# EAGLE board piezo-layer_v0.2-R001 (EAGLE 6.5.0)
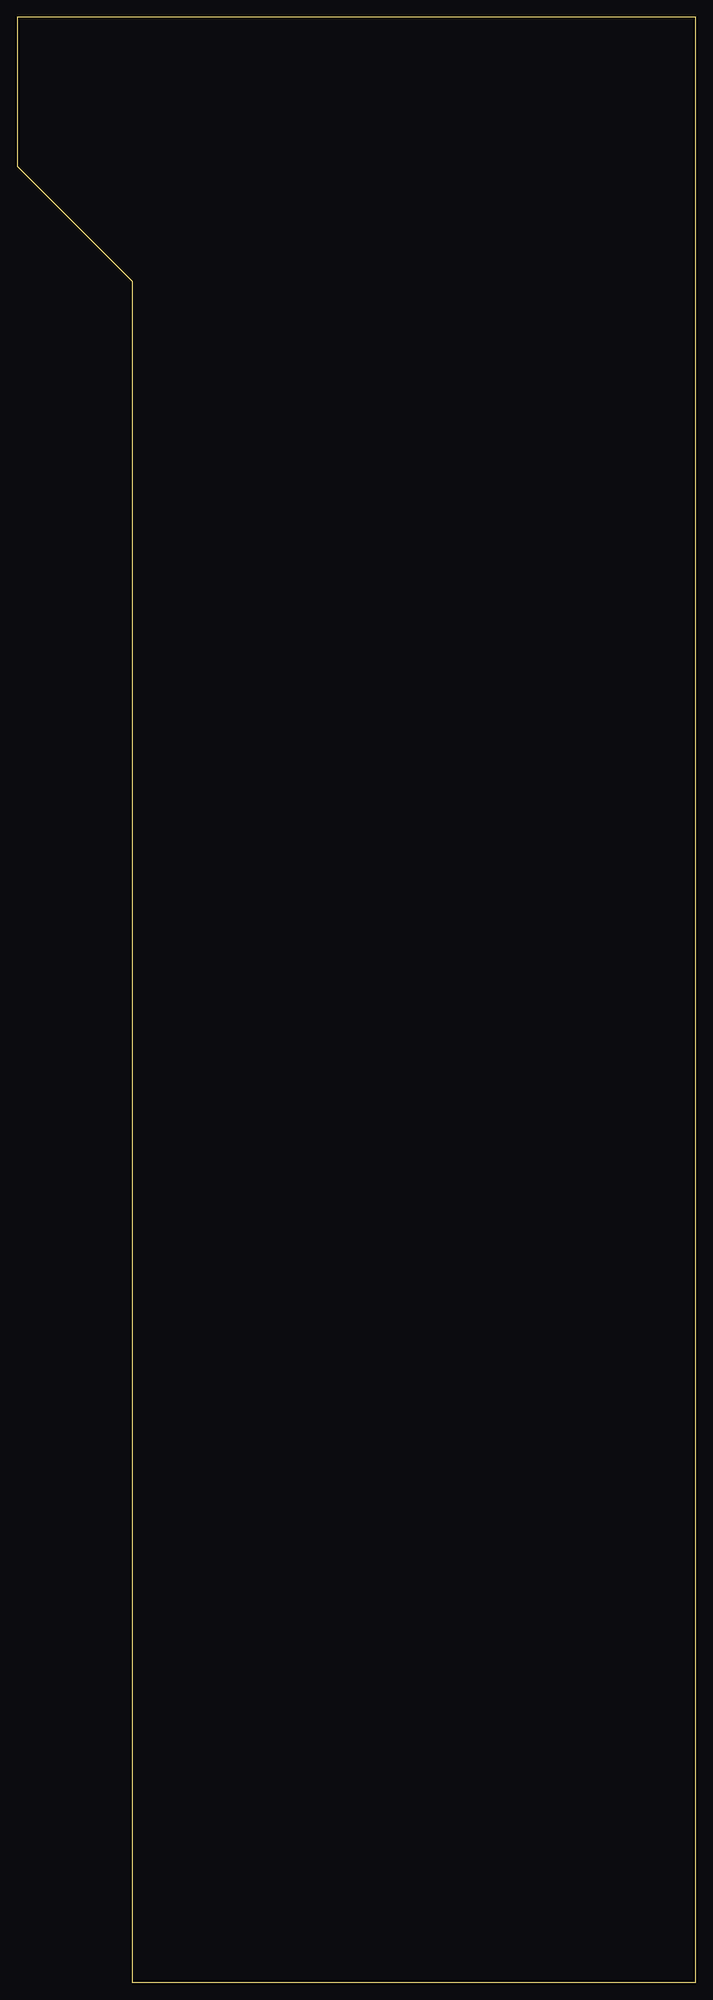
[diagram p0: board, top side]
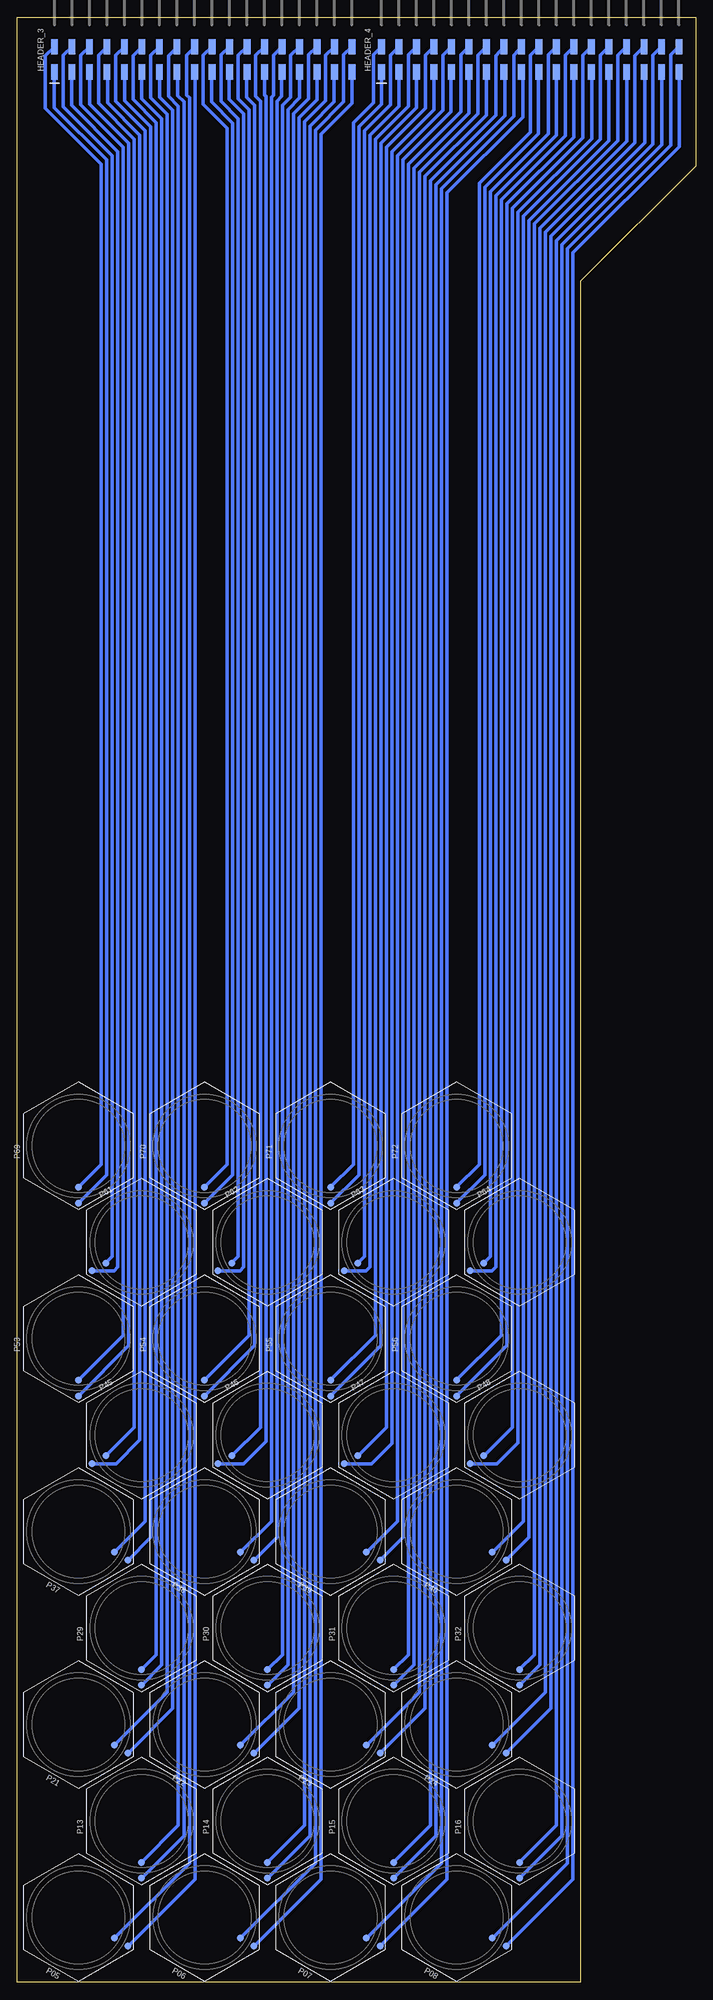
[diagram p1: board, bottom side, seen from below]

Size 98.5 x 285.2 mm. Coordinates in mm from the lower left corner, seen from the top.
Outline: 16.7,0 98.5,0 98.5,285.2 0,285.2 0,263.6 16.7,246.9 16.7,0
Copper layers (1*16): Top 0.009mm / dielectric 0.2mm / Bottom 0.018mm
Design rules "1L-0.2-0.15_0.3mm *": minimum track width 0.2mm, minimum drill 0.3mm, track to track 0.15mm, track to pad 0.15mm, pad to pad 0.15mm, via to via 0.15mm, smd to smd 0.15mm, copper to edge 0.5mm, drill to drill 1mm, minimum pad ring 10mil, minimum via ring 8mil, stop-mask expansion 4mil, vias tented up to drill 0mil, thermal gap 10mil

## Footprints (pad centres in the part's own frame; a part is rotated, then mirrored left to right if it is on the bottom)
2X18_2.54_90_SMD = smd 1 x 2.2: 1 -21.59,-1.84; 2 -21.59,1.84; 3 -19.05,-1.84; 4 -19.05,1.84; 5 -16.51,-1.84; 6 -16.51,1.84; 7 -13.97,-1.84; 8 -13.97,1.84; 9 -11.43,-1.84; 10 -11.43,1.84; 11 -8.89,-1.84; 12 -8.89,1.84; 13 -6.35,-1.84; 14 -6.35,1.84; 15 -3.81,-1.84; 16 -3.81,1.84; 17 -1.27,-1.84; 18 -1.27,1.84; 19 1.27,-1.84; 20 1.27,1.84; 21 3.81,-1.84; 22 3.81,1.84; 23 6.35,-1.84; 24 6.35,1.84; 25 8.89,-1.84; 26 8.89,1.84; 27 11.43,-1.84; 28 11.43,1.84; 29 13.97,-1.84; 30 13.97,1.84; 31 16.51,-1.84; 32 16.51,1.84; 33 19.05,-1.84; 34 19.05,1.84; 35 21.59,-1.84; 36 21.59,1.84
PIEZO-BENDER-HEX_16MM_1+_1- = smd 1 x 1: PAD1 -8.3,0; TIP1 -6,0

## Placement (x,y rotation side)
HEADER_3  HEADER_2X18-2.54_90_SMD  [2X18_2.54_90_SMD]  71.5,279.1 0 bottom
HEADER_4  HEADER_2X18-2.54_90_SMD  [2X18_2.54_90_SMD]  24,279.1 0 bottom
P05  PIEZO-BENDER-HEX_1-1  [PIEZO-BENDER-HEX_16MM_1+_1-]  89.6,9.4 150 bottom
P06  PIEZO-BENDER-HEX_1-1  [PIEZO-BENDER-HEX_16MM_1+_1-]  71.3,9.4 150 bottom
P07  PIEZO-BENDER-HEX_1-1  [PIEZO-BENDER-HEX_16MM_1+_1-]  53,9.4 150 bottom
P08  PIEZO-BENDER-HEX_1-1  [PIEZO-BENDER-HEX_16MM_1+_1-]  34.7,9.4 150 bottom
P13  PIEZO-BENDER-HEX_1-1  [PIEZO-BENDER-HEX_16MM_1+_1-]  80.45,23.4 90 bottom
P14  PIEZO-BENDER-HEX_1-1  [PIEZO-BENDER-HEX_16MM_1+_1-]  62.15,23.4 90 bottom
P15  PIEZO-BENDER-HEX_1-1  [PIEZO-BENDER-HEX_16MM_1+_1-]  43.85,23.4 90 bottom
P16  PIEZO-BENDER-HEX_1-1  [PIEZO-BENDER-HEX_16MM_1+_1-]  25.55,23.4 90 bottom
P21  PIEZO-BENDER-HEX_1-1  [PIEZO-BENDER-HEX_16MM_1+_1-]  89.6,37.4 150 bottom
P22  PIEZO-BENDER-HEX_1-1  [PIEZO-BENDER-HEX_16MM_1+_1-]  71.3,37.4 150 bottom
P23  PIEZO-BENDER-HEX_1-1  [PIEZO-BENDER-HEX_16MM_1+_1-]  53,37.4 150 bottom
P24  PIEZO-BENDER-HEX_1-1  [PIEZO-BENDER-HEX_16MM_1+_1-]  34.7,37.4 150 bottom
P29  PIEZO-BENDER-HEX_1-1  [PIEZO-BENDER-HEX_16MM_1+_1-]  80.45,51.4 90 bottom
P30  PIEZO-BENDER-HEX_1-1  [PIEZO-BENDER-HEX_16MM_1+_1-]  62.15,51.4 90 bottom
P31  PIEZO-BENDER-HEX_1-1  [PIEZO-BENDER-HEX_16MM_1+_1-]  43.85,51.4 90 bottom
P32  PIEZO-BENDER-HEX_1-1  [PIEZO-BENDER-HEX_16MM_1+_1-]  25.55,51.4 90 bottom
P37  PIEZO-BENDER-HEX_1-1  [PIEZO-BENDER-HEX_16MM_1+_1-]  89.6,65.4 150 bottom
P38  PIEZO-BENDER-HEX_1-1  [PIEZO-BENDER-HEX_16MM_1+_1-]  71.3,65.4 150 bottom
P39  PIEZO-BENDER-HEX_1-1  [PIEZO-BENDER-HEX_16MM_1+_1-]  53,65.4 150 bottom
P40  PIEZO-BENDER-HEX_1-1  [PIEZO-BENDER-HEX_16MM_1+_1-]  34.7,65.4 150 bottom
P45  PIEZO-BENDER-HEX_1-1  [PIEZO-BENDER-HEX_16MM_1+_1-]  80.45,79.4 30 bottom
P46  PIEZO-BENDER-HEX_1-1  [PIEZO-BENDER-HEX_16MM_1+_1-]  62.15,79.4 30 bottom
P47  PIEZO-BENDER-HEX_1-1  [PIEZO-BENDER-HEX_16MM_1+_1-]  43.85,79.4 30 bottom
P48  PIEZO-BENDER-HEX_1-1  [PIEZO-BENDER-HEX_16MM_1+_1-]  25.55,79.4 30 bottom
P53  PIEZO-BENDER-HEX_1-1  [PIEZO-BENDER-HEX_16MM_1+_1-]  89.6,93.4 90 bottom
P54  PIEZO-BENDER-HEX_1-1  [PIEZO-BENDER-HEX_16MM_1+_1-]  71.3,93.4 90 bottom
P55  PIEZO-BENDER-HEX_1-1  [PIEZO-BENDER-HEX_16MM_1+_1-]  53,93.4 90 bottom
P56  PIEZO-BENDER-HEX_1-1  [PIEZO-BENDER-HEX_16MM_1+_1-]  34.7,93.4 90 bottom
P61  PIEZO-BENDER-HEX_1-1  [PIEZO-BENDER-HEX_16MM_1+_1-]  80.45,107.4 30 bottom
P62  PIEZO-BENDER-HEX_1-1  [PIEZO-BENDER-HEX_16MM_1+_1-]  62.15,107.4 30 bottom
P63  PIEZO-BENDER-HEX_1-1  [PIEZO-BENDER-HEX_16MM_1+_1-]  43.85,107.4 30 bottom
P64  PIEZO-BENDER-HEX_1-1  [PIEZO-BENDER-HEX_16MM_1+_1-]  25.55,107.4 30 bottom
P69  PIEZO-BENDER-HEX_1-1  [PIEZO-BENDER-HEX_16MM_1+_1-]  89.6,121.4 90 bottom
P70  PIEZO-BENDER-HEX_1-1  [PIEZO-BENDER-HEX_16MM_1+_1-]  71.3,121.4 90 bottom
P71  PIEZO-BENDER-HEX_1-1  [PIEZO-BENDER-HEX_16MM_1+_1-]  53,121.4 90 bottom
P72  PIEZO-BENDER-HEX_1-1  [PIEZO-BENDER-HEX_16MM_1+_1-]  34.7,121.4 90 bottom

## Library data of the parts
HEADER_3 HEADER_4 = SABRe
P05-P08 P13-P16 P21-P24 P29-P32 P37-P40 P45-P48 P53-P56 P61-P64 P69-P72 = ICST

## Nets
BUS+5: HEADER_3.18 P05.TIP1
BUS+6: HEADER_3.36 P06.TIP1
BUS+7: HEADER_4.18 P07.TIP1
BUS+8: HEADER_4.36 P08.TIP1
BUS+13: HEADER_3.16 P13.TIP1
BUS+14: HEADER_3.34 P14.TIP1
BUS+15: HEADER_4.16 P15.TIP1
BUS+16: HEADER_4.34 P16.TIP1
BUS+21: HEADER_3.14 P21.TIP1
BUS+22: HEADER_3.32 P22.TIP1
BUS+23: HEADER_4.14 P23.TIP1
BUS+24: HEADER_4.32 P24.TIP1
BUS+29: HEADER_3.12 P29.TIP1
BUS+30: HEADER_3.30 P30.TIP1
BUS+31: HEADER_4.12 P31.TIP1
BUS+32: HEADER_4.30 P32.TIP1
BUS+37: HEADER_3.10 P37.TIP1
BUS+38: HEADER_3.28 P38.TIP1
BUS+39: HEADER_4.10 P39.TIP1
BUS+40: HEADER_4.28 P40.TIP1
BUS+45: HEADER_3.8 P45.TIP1
BUS+46: HEADER_3.26 P46.TIP1
BUS+47: HEADER_4.8 P47.TIP1
BUS+48: HEADER_4.26 P48.TIP1
BUS+53: HEADER_3.6 P53.TIP1
BUS+54: HEADER_3.24 P54.TIP1
BUS+55: HEADER_4.6 P55.TIP1
BUS+56: HEADER_4.24 P56.TIP1
BUS+61: HEADER_3.4 P61.TIP1
BUS+62: HEADER_3.22 P62.TIP1
BUS+63: HEADER_4.4 P63.TIP1
BUS+64: HEADER_4.22 P64.TIP1
BUS+69: HEADER_3.2 P69.TIP1
BUS+70: HEADER_3.20 P70.TIP1
BUS+71: HEADER_4.2 P71.TIP1
BUS+72: HEADER_4.20 P72.TIP1
BUS-5: HEADER_3.17 P05.PAD1
BUS-6: HEADER_3.35 P06.PAD1
BUS-7: HEADER_4.17 P07.PAD1
BUS-8: HEADER_4.35 P08.PAD1
BUS-13: HEADER_3.15 P13.PAD1
BUS-14: HEADER_3.33 P14.PAD1
BUS-15: HEADER_4.15 P15.PAD1
BUS-16: HEADER_4.33 P16.PAD1
BUS-21: HEADER_3.13 P21.PAD1
BUS-22: HEADER_3.31 P22.PAD1
BUS-23: HEADER_4.13 P23.PAD1
BUS-24: HEADER_4.31 P24.PAD1
BUS-29: HEADER_3.11 P29.PAD1
BUS-30: HEADER_3.29 P30.PAD1
BUS-31: HEADER_4.11 P31.PAD1
BUS-32: HEADER_4.29 P32.PAD1
BUS-37: HEADER_3.9 P37.PAD1
BUS-38: HEADER_3.27 P38.PAD1
BUS-39: HEADER_4.9 P39.PAD1
BUS-40: HEADER_4.27 P40.PAD1
BUS-45: HEADER_3.7 P45.PAD1
BUS-46: HEADER_3.25 P46.PAD1
BUS-47: HEADER_4.7 P47.PAD1
BUS-48: HEADER_4.25 P48.PAD1
BUS-53: HEADER_3.5 P53.PAD1
BUS-54: HEADER_3.23 P54.PAD1
BUS-55: HEADER_4.5 P55.PAD1
BUS-56: HEADER_4.23 P56.PAD1
BUS-61: HEADER_3.3 P61.PAD1
BUS-62: HEADER_3.21 P62.PAD1
BUS-63: HEADER_4.3 P63.PAD1
BUS-64: HEADER_4.21 P64.PAD1
BUS-69: HEADER_3.1 P69.PAD1
BUS-70: HEADER_3.19 P70.PAD1
BUS-71: HEADER_4.1 P71.PAD1
BUS-72: HEADER_4.19 P72.PAD1

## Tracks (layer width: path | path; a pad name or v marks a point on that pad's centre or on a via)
BUS+5
  Bottom 0.5: P05.TIP1 73.5,17.3 73.5,273.5 73.9,273.9 73.9,279.68 72.69,280.89 | 72.64,280.94 72.69,280.89 | HEADER_3.18 72.72,280.89 72.69,280.89
BUS+6
  Bottom 0.5: P06.TIP1 55.2,17.3 55.2,268.8 51.1,272.9 51.1,279.75 HEADER_3.36
BUS+7
  Bottom 0.5: P07.TIP1 36.9,17.3 36.9,260.3 26.4,270.8 26.4,279.68 HEADER_4.18
BUS+8
  Bottom 0.5: P08.TIP1 18.6,17.3 18.6,251.6 3.6,266.6 3.6,279.75 HEADER_4.36
BUS+13
  Bottom 0.5: P13.TIP1 75.1,22.75 75.1,272.3 76.5,273.7 76.5,279.62 75.18,280.94 HEADER_3.16
BUS+14
  Bottom 0.5: P14.TIP1 56.8,22.75 56.8,270 53.7,273.1 53.7,279.69 HEADER_3.34
BUS+15
  Bottom 0.5: P15.TIP1 38.5,22.75 38.5,261.5 29,271 29,279.62 HEADER_4.16
BUS+16
  Bottom 0.5: P16.TIP1 20.2,22.75 20.2,252.8 6.2,266.8 6.2,279.69 HEADER_4.34
BUS+21
  Bottom 0.5: P21.TIP1 76.7,42.1 76.7,271.1 79.1,273.5 79.1,279.69 HEADER_3.14
BUS+22
  Bottom 0.5: P22.TIP1 58.4,42.1 58.4,271.2 56.2,273.4 56.2,279.73 HEADER_3.32
BUS+23
  Bottom 0.5: P23.TIP1 40.1,42.1 40.1,262.7 31.6,271.2 31.6,279.69 HEADER_4.14
BUS+24
  Bottom 0.5: P24.TIP1 21.8,42.1 21.8,254 8.8,267 8.8,279.63 HEADER_4.32
BUS+29
  Bottom 0.5: P29.TIP1 78.3,47.55 78.3,269.9 81.7,273.3 81.7,279.63 HEADER_3.12
BUS+30
  Bottom 0.5: P30.TIP1 60,47.55 60,272.4 58.8,273.6 58.8,279.67 HEADER_3.30
BUS+31
  Bottom 0.5: P31.TIP1 41.7,47.55 41.7,263.9 34.1,271.5 34.1,279.73 HEADER_4.12
BUS+32
  Bottom 0.5: P32.TIP1 23.4,47.55 23.4,255.2 11.3,267.3 11.3,279.67 HEADER_4.30
BUS+37
  Bottom 0.5: P37.TIP1 79.9,66.9 79.9,268.7 84.2,273 84.2,279.67 HEADER_3.10
BUS+38
  Bottom 0.5: P38.TIP1 61.6,66.9 61.6,273.6 61.3,273.9 61.3,279.71 HEADER_3.28
BUS+39
  Bottom 0.5: P39.TIP1 43.3,66.9 43.3,265.1 36.7,271.7 36.7,279.67 HEADER_4.10
BUS+40
  Bottom 0.5: P40.TIP1 25,66.9 25,256.3 13.8,267.5 13.8,279.71 HEADER_4.28
BUS+45
  Bottom 0.5: P45.TIP1 81.5,80.55 81.5,267.5 86.7,272.7 86.7,279.71 HEADER_3.8
BUS+46
  Bottom 0.5: P46.TIP1 63.2,80.55 63.2,273 63.9,273.7 63.9,279.65 HEADER_3.26
BUS+47
  Bottom 0.5: P47.TIP1 44.9,80.55 44.9,266.3 39.2,272 39.2,279.71 HEADER_4.8
BUS+48
  Bottom 0.5: P48.TIP1 26.6,80.55 26.6,257.5 16.4,267.7 16.4,279.65 HEADER_4.26
BUS+53
  Bottom 0.5: P53.TIP1 83.1,93.9 83.1,266.3 89.3,272.5 89.3,279.65 HEADER_3.6
BUS+54
  Bottom 0.5: P54.TIP1 64.8,93.9 64.8,271.8 66.4,273.4 66.4,279.69 HEADER_3.24
BUS+55
  Bottom 0.5: P55.TIP1 46.5,93.9 46.5,267.5 41.7,272.3 41.7,279.75 HEADER_4.6
BUS+56
  Bottom 0.5: P56.TIP1 28.2,93.9 28.2,258.7 18.9,268 18.9,279.69 HEADER_4.24
BUS+61
  Bottom 0.5: P61.TIP1 84.7,105.35 84.7,265.1 91.8,272.2 91.8,279.69 HEADER_3.4
BUS+62
  Bottom 0.5: P62.TIP1 66.4,105.35 66.4,270.5 68.9,273 68.9,279.73 HEADER_3.22
BUS+63
  Bottom 0.5: P63.TIP1 48.1,105.35 48.1,268.7 44.3,272.5 44.3,279.69 HEADER_4.4
BUS+64
  Bottom 0.5: P64.TIP1 29.8,105.35 29.8,259.9 21.4,268.3 21.4,279.73 HEADER_4.22
BUS+69
  Bottom 0.5: P69.TIP1 86.3,118.7 86.3,263.9 94.4,272 94.4,279.63 HEADER_3.2
BUS+70
  Bottom 0.5: P70.TIP1 68,118.7 68,269.1 71.5,272.6 71.5,279.67 HEADER_3.20
BUS+71
  Bottom 0.5: P71.TIP1 49.7,118.7 49.7,269.9 46.8,272.8 46.8,279.73 HEADER_4.2
BUS+72
  Bottom 0.5: P72.TIP1 31.4,118.7 31.4,261.1 24,268.5 24,279.67 HEADER_4.20
BUS-5
  Bottom 0.5: P05.PAD1 72.7,14.96 72.7,277.2 | 72.64,277.26 72.7,277.2 | 72.7,277.2 72.76,277.26 HEADER_3.17
BUS-6
  Bottom 0.5: P06.PAD1 54.4,14.96 54.4,268.2 49.9,272.7 HEADER_3.35
BUS-7
  Bottom 0.5: P07.PAD1 36.1,14.96 36.1,259.7 25.1,270.7 25.1,277.22 HEADER_4.17
BUS-8
  Bottom 0.5: P08.PAD1 17.8,14.96 17.8,251 2.4,266.4 HEADER_4.35
BUS-13
  Bottom 0.5: P13.PAD1 74.3,21.25 74.3,272.9 75.2,273.8 75.2,277.15 | 75.18,277.26 75.2,277.24 75.2,277.15 | HEADER_3.15 75.2,277.15
BUS-14
  Bottom 0.5: P14.PAD1 56,21.25 56,269.4 52.5,272.9 52.5,277.21 HEADER_3.33
BUS-15
  Bottom 0.5: P15.PAD1 37.7,21.25 37.7,260.9 27.7,270.9 27.7,277.24 HEADER_4.15
BUS-16
  Bottom 0.5: P16.PAD1 19.4,21.25 19.4,252.2 4.9,266.7 4.9,277.21 HEADER_4.33
BUS-21
  Bottom 0.5: P21.PAD1 75.9,39.76 75.9,271.7 77.8,273.6 77.8,277.21 HEADER_3.13
BUS-22
  Bottom 0.5: P22.PAD1 57.6,39.76 57.6,270.6 55,273.2 HEADER_3.31
BUS-23
  Bottom 0.5: P23.PAD1 39.3,39.76 39.3,262.1 30.4,271 30.4,277.21 HEADER_4.13
BUS-24
  Bottom 0.5: P24.PAD1 21,39.76 21,253.4 7.4,267 7.4,277.17 HEADER_4.31
BUS-29
  Bottom 0.5: P29.PAD1 77.5,46.05 77.5,270.5 80.4,273.4 HEADER_3.11
BUS-30
  Bottom 0.5: P30.PAD1 59.2,46.05 59.2,271.8 57.5,273.5 57.5,277.23 HEADER_3.29
BUS-31
  Bottom 0.5: P31.PAD1 40.9,46.05 40.9,263.3 32.9,271.3 HEADER_4.11
BUS-32
  Bottom 0.5: P32.PAD1 22.6,46.05 22.6,254.6 10,267.2 10,277.23 HEADER_4.29
BUS-37
  Bottom 0.5: P37.PAD1 79.1,64.56 79.1,269.3 82.9,273.1 82.9,277.23 HEADER_3.9
BUS-38
  Bottom 0.5: P38.PAD1 60.8,64.56 60.8,273 60.1,273.7 60.1,277.23 HEADER_3.27
BUS-39
  Bottom 0.5: P39.PAD1 42.5,64.56 42.5,264.5 35.5,271.5 35.5,277.19 HEADER_4.9
BUS-40
  Bottom 0.5: P40.PAD1 24.2,64.56 24.2,255.7 12.6,267.3 12.6,277.23 HEADER_4.27
BUS-45
  Bottom 0.5: P45.PAD1 84.15,75.25 80.7,78.7 80.7,268.1 85.4,272.8 85.4,277.19 HEADER_3.7
BUS-46
  Bottom 0.5: P46.PAD1 65.65,75.25 62.4,78.5 62.4,273.7 62.6,273.9 HEADER_3.25
BUS-47
  Bottom 0.5: P47.PAD1 47.05,75.25 44.1,78.2 44.1,265.7 38,271.8 38,277.23 HEADER_4.7
BUS-48
  Bottom 0.5: P48.PAD1 28.85,75.25 25.8,78.3 25.8,256.9 15.1,267.6 HEADER_4.25
BUS-53
  Bottom 0.5: P53.PAD1 82.3,92.4 82.3,266.9 88,272.6 HEADER_3.5
BUS-54
  Bottom 0.5: P54.PAD1 64,92.4 64,272.4 65.2,273.6 65.2,277.21 HEADER_3.23
BUS-55
  Bottom 0.5: P55.PAD1 45.7,92.4 45.7,266.9 40.5,272.1 HEADER_4.5
BUS-56
  Bottom 0.5: P56.PAD1 27.4,92.4 27.4,258.1 17.7,267.8 17.7,277.21 HEADER_4.23
BUS-61
  Bottom 0.5: P61.PAD1 84.45,103.25 83.9,103.8 83.9,265.7 90.6,272.4 90.6,277.21 HEADER_3.3
BUS-62
  Bottom 0.5: P62.PAD1 66.15,103.25 65.6,103.8 65.6,271.2 67.7,273.3 HEADER_3.21
BUS-63
  Bottom 0.5: P63.PAD1 47.85,103.25 47.3,103.8 47.3,268.1 43.1,272.3 43.1,277.21 HEADER_4.3
BUS-64
  Bottom 0.5: P64.PAD1 29.55,103.25 29,103.8 29,259.3 20.2,268.1 HEADER_4.21
BUS-69
  Bottom 0.5: P69.PAD1 85.5,117.2 85.5,264.5 93.1,272.1 HEADER_3.1
BUS-70
  Bottom 0.5: P70.PAD1 67.2,117.2 67.2,269.8 70.3,272.9 70.3,277.19 HEADER_3.19
BUS-71
  Bottom 0.5: P71.PAD1 48.9,117.2 48.9,269.3 45.6,272.6 HEADER_4.1
BUS-72
  Bottom 0.5: P72.PAD1 30.6,117.2 30.6,260.5 22.8,268.3 22.8,277.19 HEADER_4.19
